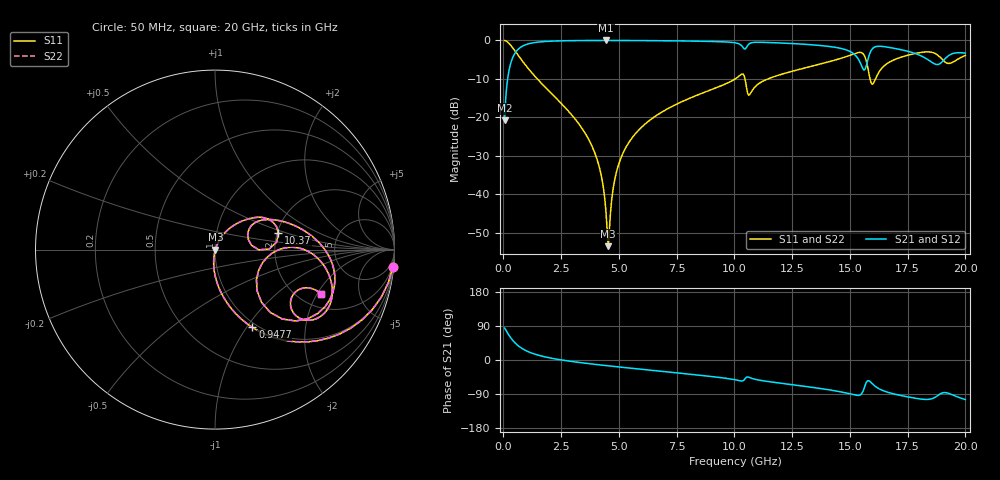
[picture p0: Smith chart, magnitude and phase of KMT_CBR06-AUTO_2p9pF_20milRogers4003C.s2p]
! Data measured by Modelithics Inc. support@modelithics.com 813-866-6335
! KEMET CBR06-AUTO 2.9pF, Pad Width= 0.851mm, Pad Length= 0.64mm, Pad Gap= 0.62mm, 20mil Rogers 4003C substrate Data, January 2022
# hz S ma R 50
! 2 Port Network Data from SP1.SP block
! freq  magS11  angS11  magS21  angS21  magS12  angS12  magS22  angS22
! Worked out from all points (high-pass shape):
!   401 points, 50 MHz to 20 GHz, reference 50 ohm
!   highest |S21| = -0.02 dB at 4.439 GHz (marker M1); lowest = -20.7 dB at 50 MHz (marker M2)
!   |S21| within 3 dB of the highest: 535.8 MHz to 15.05 GHz (14.51 GHz wide, 186 % of centre); 15.89 GHz to 17.62 GHz (1.733 GHz wide, 10.3 % of centre)
!   lowest |S11| = -53.4 dB at 4.539 GHz (marker M3), VSWR 1.00, Z = 50.2 - j0.051 ohm
!   |S11| at or under -10 dB: 1.465 GHz to 10.03 GHz (8.567 GHz wide, 149 % of centre); 10.46 GHz to 11.45 GHz (993.3 MHz wide, 9.07 % of centre); 15.87 GHz to 16.11 GHz (236.1 MHz wide, 1.48 % of centre)
!   |S22| runs from -53.4 to 0.0 dB; largest |S21 - S12| = 0
!   S11 on the Smith chart (normalised r, x): 50 MHz: 1, -21; 947.8 MHz: 0.94, -1.06; 10.37 GHz: 2.03, +0.43; 20 GHz: 2.59, -2.14
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5e7  0.9957 -5.4  0.09182 84.5  0.09182 84.5  0.9957 -5.4
3.4925e8  0.8389 -34.1  0.5433 55.8  0.5433 55.8  0.8389 -34.1
9.4775e8  0.4806 -64.4  0.8757 25.5  0.8757 25.5  0.4806 -64.4
3.391625e9  0.07293 -95.9  0.9954 -7.4  0.9954 -7.4  0.07293 -95.9
4.089875e9  0.02627 -98.0  0.9975 -12.4  0.9975 -12.4  0.02627 -98.0
4.289375e9  0.0144 -95.5  0.9977 -13.8  0.9977 -13.8  0.0144 -95.5
4.439e9  0.005972 -84.1  0.9977 -14.8  0.9977 -14.8  0.005972 -84.1
4.53875e9  0.002135 -13.8  0.9977 -15.4  0.9977 -15.4  0.002135 -13.8
4.838e9  0.01664 65.0  0.9975 -17.4  0.9975 -17.4  0.01664 65.0
5.187125e9  0.03496 66.6  0.9969 -19.6  0.9969 -19.6  0.03496 66.6
6.73325e9  0.1113 59.4  0.9908 -29.2  0.9908 -29.2  0.1113 59.4
1.0025e10  0.3152 34.7  0.9308 -52.0  0.9308 -52.0  0.3152 34.7
1.037412e10  0.3655 14.5  0.8103 -54.8  0.8103 -54.8  0.3655 14.5
1.067338e10  0.2001 24.3  0.9165 -46.7  0.9165 -46.7  0.2001 24.3
1.336662e10  0.4638 16.7  0.8761 -72.1  0.8761 -72.1  0.4638 16.7
1.526188e10  0.6824 -12.2  0.6281 -92.8  0.6281 -92.8  0.6824 -12.2
1.566088e10  0.6003 -41.5  0.4225 -66.4  0.4225 -66.4  0.6003 -41.5
1.601e10  0.2746 -15.6  0.7983 -64.9  0.7983 -64.9  0.2746 -15.6
1.670825e10  0.5218 -1.2  0.8094 -86.4  0.8094 -86.4  0.5218 -1.2
1.870325e10  0.6733 -35.4  0.4903 -97.9  0.4903 -97.9  0.6733 -35.4
1.915212e10  0.5152 -35.4  0.5904 -86.2  0.5904 -86.2  0.5152 -35.4
2e10  0.6382 -22.6  0.6831 -104.4  0.6831 -104.4  0.6382 -22.6
